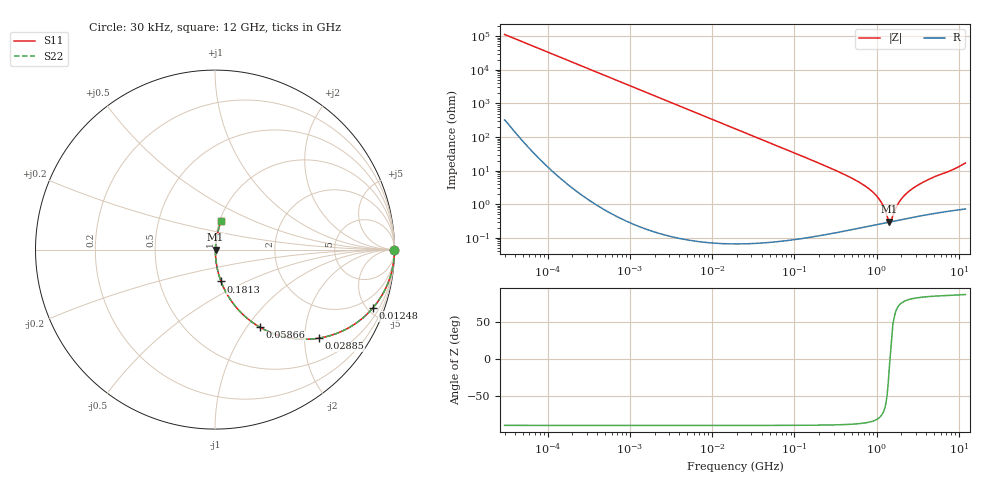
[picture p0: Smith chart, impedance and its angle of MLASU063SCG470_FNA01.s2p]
! MLASU063SCG470_FNA01  S-PARAMETER MODEL  ( General Type )
! Model Generated by TAIYO YUDEN Corporation (http://www.ty-top.com)
! Version 2.0
! TAIYO YUDEN Control No. 141022
! Copyright(c) 2013 TAIYO YUDEN CO.,LTD. All Rights Reserved.
! Product Description (link to TY-COMPAS)
! https://ds.yuden.co.jp/TYCOMPAS/or/detail?pn=MLASU063SCG470JFNA01&u=M
! Products Name : Multilayer Ceramic Capacitors
! Characteristics :
!  Capacitance : 47 pF , Rated Voltage : 50V , TCC : CG / C0G
!  Case Size : 0.6 x 0.3 / 0.024 x 0.012 [mm/inch] , Thickness : 0.3 / 0.012 [mm/inch]
!  (Conditions: Temperature = 25 degC , DC Bias Current/Voltage = 0A / 0V)
! External Node Assignments :
!  1  o---| |---o  2
! GND o---------o GND
! Frequency Range : 0.03MHz  -  12000MHz  [ 401 STEP ]
# MHz S RI R 50
! Freq[MHz].  S11 Real  S11 Imag  S21 Real  S21 Imag  S12 Real  S12 Imag  S22 Real  S22 Imag
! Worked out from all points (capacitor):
!   401 points, 30 kHz to 12 GHz, reference 50 ohm
!   read as one part in series: C = 47 pF near 32 kHz
!   lowest |Z| = 302 mohm at 1.428 GHz (marker M1)
!   series resonance near 1.455 GHz, so ESL is about 250 pH
!   S11 on the Smith chart (normalised r, x): 30 kHz: open; 12.48 MHz: 1.00, -5.43; 28.85 MHz: 1.00, -2.35; 58.66 MHz: 1.00, -1.15; 181.3 MHz: 1.00, -0.37; 12 GHz: 1.01, +0.34
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0.03  1 -0.000886  3.31e-06 0.000886  3.31e-06 0.000886  1 -0.000886
0.260295  0.9999 -0.00769  6.02e-05 0.00769  6.02e-05 0.00769  0.9999 -0.00769
2.258455  0.9956 -0.0664  0.00443 0.0664  0.00443 0.0664  0.9956 -0.0664
5.571287  0.9736 -0.1602  0.0264 0.1602  0.0264 0.1602  0.9736 -0.1602
12.47626  0.8804 -0.3244  0.1196 0.3244  0.1196 0.3244  0.8804 -0.3244
18.97367  0.7609 -0.4263  0.2391 0.4263  0.2391 0.4263  0.7609 -0.4263
28.85481  0.5791 -0.4934  0.4209 0.4934  0.4209 0.4934  0.5791 -0.4934
58.65857  0.2496 -0.4321  0.7504 0.4321  0.7504 0.4321  0.2496 -0.4321
95.14999  0.1121 -0.3143  0.8879 0.3143  0.8879 0.3143  0.1121 -0.3143
164.6252  0.0405 -0.1946  0.9595 0.1946  0.9595 0.1946  0.0405 -0.1946
181.3476  0.0337 -0.1774  0.9663 0.1774  0.9663 0.1774  0.0337 -0.1774
462.0203  0.00597 -0.0652  0.994 0.0652  0.994 0.0652  0.00597 -0.0652
799.3715  0.00306 -0.0291  0.9969 0.0291  0.9969 0.0291  0.00306 -0.0291
970.0175  0.0028 -0.019  0.9972 0.019  0.9972 0.019  0.0028 -0.019
1103.571  0.00276 -0.0126  0.9972 0.0126  0.9972 0.0126  0.00276 -0.0126
1428.372  0.00296 -0.000571  0.997 0.000571  0.997 0.000571  0.00296 -0.000571
1523.532  0.00305 0.00162  0.9969 -0.00162  0.9969 -0.00162  0.00305 0.00162
1790.1  0.00338 0.00887  0.9966 -0.00887  0.9966 -0.00887  0.00338 0.00887
1971.936  0.00364 0.0133  0.9964 -0.0133  0.9964 -0.0133  0.00364 0.0133
2635.962  0.0047 0.0269  0.9953 -0.0269  0.9953 -0.0269  0.0047 0.0269
4275.791  0.00783 0.0536  0.9922 -0.0536  0.9922 -0.0536  0.00783 0.0536
12000  0.0341 0.1614  0.9659 -0.1614  0.9659 -0.1614  0.0341 0.1614
